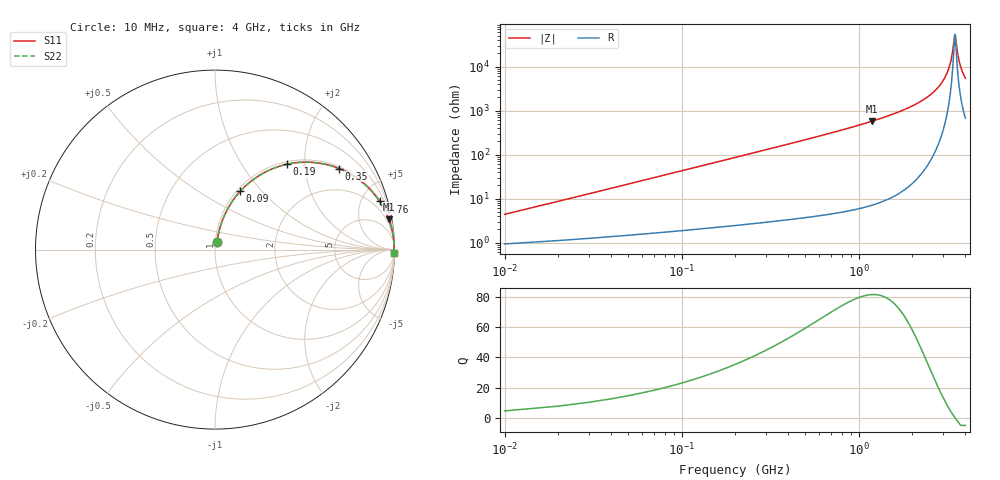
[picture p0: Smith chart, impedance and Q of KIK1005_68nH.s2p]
!version-1
!date-01.2023
!Series
# MHz S RI R 50
!Freq ReS11 ImS11 ReS21 ImS21 ReS12 ImS12 ReS22 ImS22
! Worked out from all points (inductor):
!   400 points, 10 MHz to 4 GHz, reference 50 ohm
!   read as one part in series: L = 68 nH near 30 MHz
!   highest Q = 81.3 at 1.19 GHz (marker M1), where L = 76.9 nH
!   self-resonance near 3.49 GHz
!   S11 on the Smith chart (normalised r, x): 10 MHz: 1.02, +0.09; 90 MHz: 1.04, +0.77; 190 MHz: 1.05, +1.63; 350 MHz: 1.06, +3.02; 760 MHz: 1.09, +6.82; 4 GHz: open
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10  0.011 0.0419  0.989 -0.0419  0.989 -0.0419  0.011 0.0419
20  0.018 0.083  0.982 -0.083  0.982 -0.083  0.018 0.083
40  0.0407 0.1618  0.9593 -0.1618  0.9593 -0.1618  0.0407 0.1618
90  0.1404 0.3249  0.8596 -0.3249  0.8596 -0.3249  0.1404 0.3249
190  0.4017 0.4758  0.5983 -0.4758  0.5983 -0.4758  0.4017 0.4758
350  0.6918 0.4516  0.3082 -0.4516  0.3082 -0.4516  0.6918 0.4516
490  0.8161 0.379  0.1839 -0.379  0.1839 -0.379  0.8161 0.379
680  0.8977 0.2958  0.1023 -0.2958  0.1023 -0.2958  0.8977 0.2958
760  0.9176 0.2681  0.0824 -0.2681  0.0824 -0.2681  0.9176 0.2681
1190  0.9687 0.168  0.0313 -0.168  0.0313 -0.168  0.9687 0.168
1340  0.9766 0.1452  0.0234 -0.1452  0.0234 -0.1452  0.9766 0.1452
2010  0.9926 0.0772  0.00736 -0.0772  0.00736 -0.0772  0.9926 0.0772
2670  0.9973 0.0363  0.00274 -0.0363  0.00274 -0.0363  0.9973 0.0363
3090  0.9981 0.0164  0.00187 -0.0164  0.00187 -0.0164  0.9981 0.0164
3230  0.9982 0.0105  0.00179 -0.0105  0.00179 -0.0105  0.9982 0.0105
3340  0.9982 0.00603  0.00178 -0.00603  0.00178 -0.00603  0.9982 0.00603
3470  0.9982 0.000932  0.00183 -0.000932  0.00183 -0.000932  0.9982 0.000932
3500  0.9981 -0.000217  0.00185 0.000217  0.00185 0.000217  0.9981 -0.000217
3610  0.9981 -0.00434  0.00195 0.00434  0.00195 0.00434  0.9981 -0.00434
3690  0.998 -0.00727  0.00204 0.00727  0.00204 0.00727  0.998 -0.00727
3820  0.9978 -0.0119  0.00224 0.0119  0.00224 0.0119  0.9978 -0.0119
4000  0.9974 -0.0181  0.00257 0.0181  0.00257 0.0181  0.9974 -0.0181
